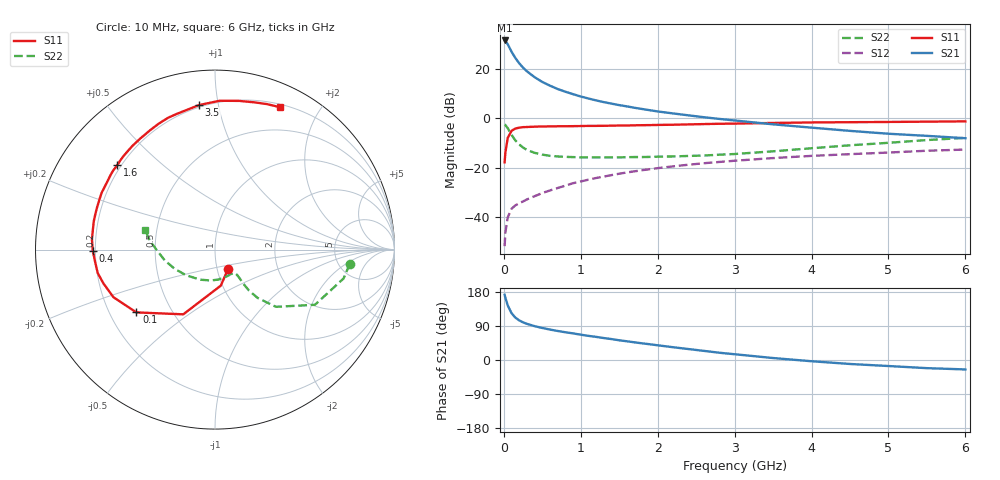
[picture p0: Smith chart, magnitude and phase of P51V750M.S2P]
! SIEMENS Small Signal Semiconductors
! BFP183
! Si NPN RF Bipolar Junction Transistor in SOT143
! VCE = 1.75 V  IC = 50 mA
! Common Emitter S-Parameters:  March  1996
# GHz  S  MA  R  50
!  f  S11  S21  S12  S22
! GHz  MAG  ANG  MAG  ANG  MAG  ANG  MAG  ANG
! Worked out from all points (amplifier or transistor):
!   36 points, 10 MHz to 6 GHz, reference 50 ohm
!   highest |S21| = 31.6 dB at 10 MHz (marker M1)
!   |S21| within 3 dB of that: start of sweep to 74.53 MHz
!   unconditionally stable (mu >= 1): start of sweep to 27.41 MHz; 208.2 MHz to end of sweep
!   at 250 MHz: K = 1.11, MAG = 25.1 dB, |S12| = -33.6 dB
!   at 1.4 GHz: K = 1.65, MAG = 9.7 dB, |S12| = -22.9 dB
!   at 6 GHz: K = 1.29, MAG = -0.9 dB, |S12| = -12.6 dB
!   S11 on the Smith chart (normalised r, x): 10 MHz: 1.13, -0.25; 100 MHz: 0.31, -0.32; 400 MHz: 0.19, -0.00; 1.6 GHz: 0.19, +0.36; 3.5 GHz: 0.19, +0.88; 6 GHz: 0.23, +1.53
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0.01  0.1294 -55.6  37.84 172.1  0.0026 70.1  0.7549 -6.1
0.02  0.2032 -80.8  37.19 164.4  0.0049 69.0  0.7339 -12.7
0.05  0.4016 -116.1  31.79 144.3  0.0099 61.3  0.6362 -28.9
0.1  0.5607 -141.4  22.43 123.5  0.0149 49.3  0.4657 -43.2
0.15  0.625 -154.9  16.71 111.8  0.0174 45.8  0.3588 -48.6
0.2  0.6498 -163.2  13.06 104.5  0.0193 46.5  0.2967 -50.3
0.25  0.6664 -168.7  10.65 99.3  0.0209 47.5  0.2575 -50.3
0.3  0.6706 -173.6  8.996 95.4  0.023 50.3  0.2308 -49.9
0.4  0.6811 -179.5  6.837 89.3  0.0267 53.8  0.2014 -49.1
0.5  0.688 175.3  5.466 84.5  0.0309 55.4  0.1851 -49.0
0.6  0.6893 170.8  4.606 80.3  0.0349 57.7  0.1749 -49.3
0.7  0.6937 166.8  3.934 76.6  0.0391 59.2  0.1699 -50.2
0.9  0.6979 160.3  3.096 70.2  0.0489 60.4  0.1651 -53.6
1.1  0.7064 153.5  2.531 63.7  0.0577 60.4  0.1624 -57.9
1.3  0.7092 147.9  2.137 57.9  0.0666 59.7  0.1626 -63.3
1.6  0.7195 139.1  1.753 49.4  0.0808 58.0  0.1643 -71.7
2.2  0.7461 123.8  1.263 33.7  0.1072 52.4  0.1701 -92.1
2.8  0.7798 109.5  0.978 19.2  0.1315 46.0  0.1845 -114.3
3.5  0.8103 96.3  0.76 5.2  0.1577 38.9  0.2161 -138.9
4.5  0.8391 80.9  0.56 -10.5  0.1893 28.4  0.2863 -167.9
5.5  0.8607 70.4  0.444 -21.5  0.222 19.0  0.3651 172.5
6  0.872 65.5  0.398 -24.9  0.2345 13.8  0.4046 164.3
